(* Logix 5000 AddOnInstructionDefinition export Banner_Q4X_Param_v4; software revision 33.00 *)

TYPE Banner_IOL_Port_v4 :   // UDT that has all of the data items necessary to communicate with a specific Port on a IO-Link Master
STRUCT
   Port_Controlled : INT;   // Each bit represents a port on an IO-Link Master. Set to 1 to tell AOI to control that port.
   Port_Activate : INT;   // Each bit represents a port on an IO-Link Master. When ON that port will process any commands in queue.
   Port_Read : INT;   // Each bit represents a port on an IO-Link Master. Used to determine when device AOI has requested a Read command.
   Port_Write : INT;   // Each bit represents a port on an IO-Link Master. Used to determine when device AOI has requested a Write command.
   Port_RW_Complete : INT;   // Each bit represents a port on an IO-Link Master. Tells device AOI that Read or Write request has been completed.
   Port_Device_Read : INT;
   Data_Transfer : SINT[190];   // Array to transfer data from IO-Master to device AOIs.
END_STRUCT
END_TYPE

TYPE Banner_Q4X_RD_v4 :   // UDT that stores the Write Data for a Q4X.
STRUCT
   Master_Cycle_Time : INT;
   Min_Cycle_Time : INT;
   M_Sequence_Capability : INT;
   IO_Link_Version_ID : INT;
   Process_Data_Input_Length : INT;
   Process_Data_Output_Length : INT;
   Combined_Vendor_ID : DINT;   // IO-Link Vendor ID
   Vendor_ID1 : INT;
   Vendor_ID2 : INT;
   Combined_Device_ID : DINT;   // IO-Link Device ID
   Device_ID1 : INT;
   Device_ID2 : INT;
   Device_ID3 : INT;
   Serial_Number : STRING;
   Teach_State : SINT;   // 0 =IDLE, 1 = SP1 Success, 4 = Wait for Command, 5 = Busy, 7 = Error
   SP1_TP1 : SINT;   // 0 = not taught or unsuccessful, 1 = successfully taught
   SP2_TP2 : SINT;   // 0 = not taught or unsuccessful, 1 = successfully taught
   Measurement_Value : DINT;   // Measurement value in .1 mm. Dual mode the value is in percent match to taught object.
   Excess_Gain_Percent : DINT;   // Excess gain expressed as a percentage of minimum signal strength.
   Stability : INT;   // 0 = No target exists, 1 = Marginal or multiple peaks, 2 = Stable
   Multiple_Peak_State : INT;   // 0 = Multiple peaks not present, 1 = Multiple peaks present
   Laser_Fault_Status : INT;   // 0 = Not present, 1 Laser fault present
   BDC1_Totalizer_Counts : DINT;   // Number of totalizer edges seen on BDC1. Range: 0 to 65535.
   BDC2_Totalizer_Counts : DINT;   // Number of totalizer edges seen on BDC2. Range: 0 to 65535.
   Display_String : STRING;   // String currently being displayed on the LED display of the sensor
END_STRUCT
END_TYPE

TYPE Banner_Q4X_v4 :   // All of the parameters for a Q4X.
STRUCT
   Initial_Global_Read : BOOL;   // Determines if all of the IO-Link data has been read into the PLC yet
   Command : INT;   // Value placed in here will activate a read or write to a specifc IO-Link Index
   Read_Data : Banner_Q4X_RD_v4;   // Read Only Data
   Write_Data : Banner_Q4X_WD_v4;   // Write Data
   Archive : Banner_Q4X_WD_v4;   // Archive of Write Data. Used to determine when data needs to be updated in the IO-Link Master.
   Reset : BOOL;   // Resets AOI. This will force a complete parameter read of the sensor.
END_STRUCT
END_TYPE

TYPE Banner_Q4X_WD_v4 :   // UDT that stores the Write Data for a Q4X.
STRUCT
   System_Command : INT;   // See IODD file for list of commands that can be activated via the System Command interface
   Parameter_Access_Lock : SINT;   // Write access to all parameters is prohibited while value is 1. Only this parameter can be adjusted when value is 1.
   Data_Storage_Lock : SINT;   // Automatic data storage is disabled when this value is equal to 1. Read access is not affected.
   Local_Parameterization_Lock : SINT;   // Parameterization via local control elements on device is disabled.
   Local_User_Interface_Lock : SINT;   // Operation of local user interface is disabled.
   Teach_Channel : INT;   // 0 = Default, 1 = BDC1, 2 = BDC2
   BDC1_Setpoint_SP1 : DINT;   // Switch point value in .1 mm increments. Range: varies depending on sensor.
   BDC1_Setpoint_SP2 : DINT;   // In FGS mode defines second switching point parameter. Range: varies depending on sensor.
   BDC1_Swithpoint_Logic : INT;   // 0 = Light Operate, 1 = Dark Operate
   BDC1_BDC_Mode : INT;   // 1 = 1-Pt BGS, 128 = 2-Pt, 129 = Dynamic, 130 = Window or FGS, 131 = Dual
   BDC1_Hysteresis : DINT;   // Should always be 0
   BDC2_Setpoint_SP1 : DINT;   // Switch point value in .1 mm increments. Range: varies depending on sensor.
   BDC2_Setpoint_SP2 : DINT;   // In FGS mode defines second switching point parameter. Range: varies depending on sensor.
   BDC2_Switchpoint_Logic : INT;   // 0 = Light Operate, 1 = Dark Operate
   BDC2_BDC_Mode : INT;   // 1 = 1-Pt BGS, 128 = 2-Pt, 129 = Dynamic, 130 = Window or FGS, 131 = Dual
   BDC2_Hysteresis : DINT;   // Should always be 0
   Response_Speed : INT;   // 0 = 1.5 ms, 1 = 3 ms, 2 = 10 ms, 3 = 25 ms, 4 = 50 ms
   Gain : INT;   // 0 = High excess gain mode, 1 = Standard excess gain mode
   Secondary_Output_Function : INT;   // 0 = Independent Output, 1 = Complimentary Output, 2 = Remote Teach Input, 3 = Laser Off, 4 = Laser On, 5 = Master, 6 = Slave, 7 = Pulse Frequency Modulation
   Zero_Reference_Location : INT;   // 0 = Near, 1 = Far
   Shift_Zero_Reference_After_Teach : INT;   // 0 = On, 1 = Off
   Display_Read : INT;   // 0 = On, 1 = On Inverted, 2 Off, 3 Off Inverted
   Pushbutton_Lockout : INT;   // 0 = No lockout, 1 = Pushbuttons locked, 2 = Operator Lockout
   IOL_Filter_Time : DINT;   // Time to average IOL process data measurement between updates. Range 0 to 65535 ms.
   BDC1_Delay_Mode : INT;   // 0 = Disabled, 1 = On - Off Delay, 2 = Oneshot, 3 = Totalizer
   BDC1_Delay_Timer1 : DINT;   // Time in 1 ms increments for 1.5 and 3 ms response speeds. Time in 10 ms for all other response speeds. If totalizer is selected value is in counts. Range 0 to 9999 ms.
   BDC1_Delay_Timer2 : DINT;   // Off Delay time in 1 ms increments for 1.5 and 3 ms response speeds. Time in 10 ms for all other response speeds. If totalizer is selected value is in counts. Range 0 to 9999 ms.
   BDC1_Teach_Offset_Mode : INT;   // 0 = Auto, 1 = User Selected
   BDC1_Teach_Offset : DINT;   // Teach Offset Mode must be in in User Selected for this to work. After a FGS or BGS teach the setpoint will be offset by the value stored in the parameter. Range: Values vary by sensor.
   BDC1_FGS_Window_Size : DINT;   // Teach Offset Mode must be in User Selected for this to work. Parameter sets the FGS window size. This value create a window +/- the value. Range: Values vary by sensor.
   BDC1_Auto_Thresholding : INT;   // 0 = On, 1 = Off, 2 = High Speed (Dual Mode Only)
   BDC2_Delay_Mode : INT;   // 0 = Disabled, 1 = On - Off Delay, 2 = Oneshot, 3 = Totalizer
   BDC2_Delay_Timer1 : DINT;   // Time in 1 ms increments for 1.5 and 3 ms response speeds. Time in 10 ms for all other response speeds. If totalizer is selected value is in counts. Range 0 to 9999 ms.
   BDC2_Delay_Timer2 : DINT;   // Off Delay time in 1 ms increments for 1.5 and 3 ms response speeds. Time in 10 ms for all other response speeds. If totalizer is selected value is in counts. Range 0 to 9999 ms.
   BDC2_Teach_Offset_Mode : INT;   // 0 = Auto, 1 = User Selected
   BDC2_Teach_Offset : DINT;   // Teach Offset Mode must be in in User Selected for this to work. After a FGS or BGS teach the setpoint will be offset by the value stored in the parameter. Range: Values vary by sensor.
   BDC2_FGS_Window_Size : DINT;   // Teach Offset Mode must be in User Selected for this to work. Parameter sets the FGS window size. This value create a window +/- the value. Range: Values vary by sensor.
   BDC2_Auto_Thresholding : INT;   // 0 = On, 1 = Off, 2 = High Speed (Dual Mode Only)
   Near_Frequency : DINT;   // Frequency corresponding to a target at the near limit of the sensing range. Range 10 to 45000 Hz.
   Far_Frequency : DINT;   // Frequency corresponding to a target at the far limit of the sensing range. Range 10 to 45000 Hz.
END_STRUCT
END_TYPE

ADD_ON_INSTRUCTION Banner_Q4X_Param_v4   (* revision 4.2, vendor Banner Engineering *)
// AOI to read and write parameter data to an IO-Link Q4X.
// Revision note:
// Fixed an issue with the Device ID parameter.
VAR_IN_OUT
   Q4X : Banner_Q4X_v4; {required}
   Port_Data : Banner_IOL_Port_v4; {required}
END_VAR
VAR_INPUT
   Port : INT; {required}   // Enter the Port number that this AOI is to work with.
END_VAR
VAR
   Local_Control : DINT; {access None}
   Global_Read_Command_Value : INT; {access None}
   Global_Write_Command_Value : INT; {access None}
   Command_Being_Processed : BOOL; {access None}
   Update_Archive : BOOL; {access None}
   Index_Write_Inprocess : INT; {access None}
   Index_Write_Control : INT; {access None}
   Temp_Excess_Gain : DINT[2]; {access None}
   Inprocess_Index : DINT; {access None}
END_VAR

ROUTINE Logic   (* ladder *)
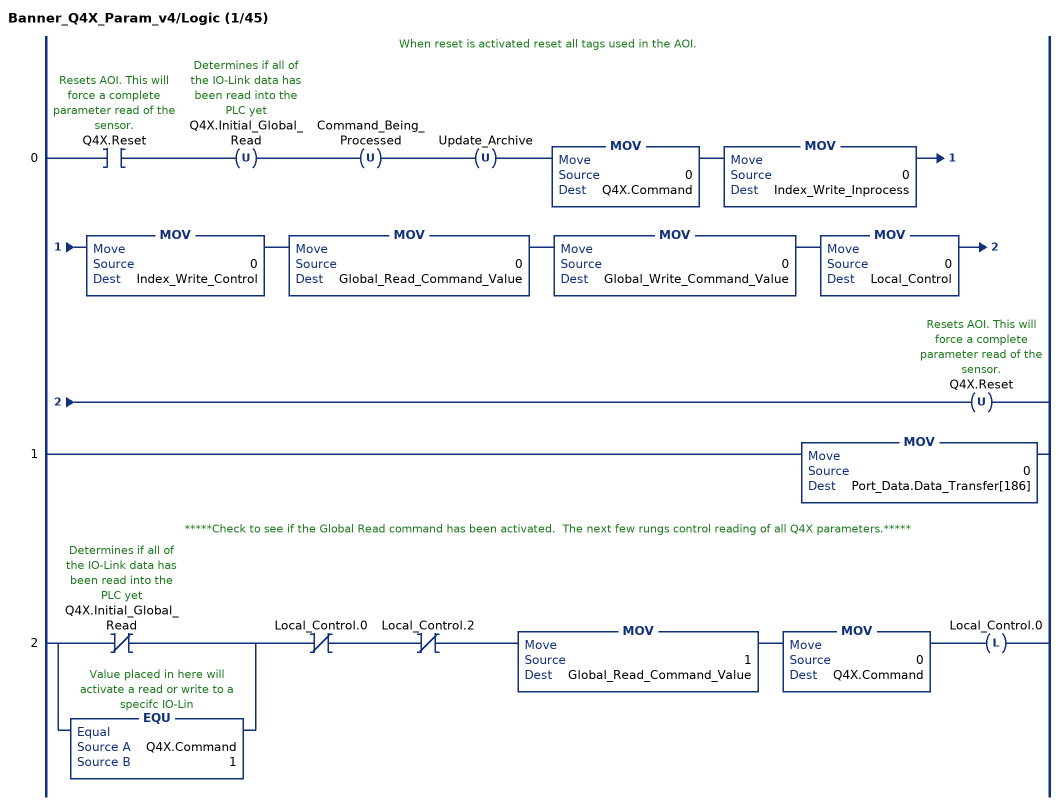
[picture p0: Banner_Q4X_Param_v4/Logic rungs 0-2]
   // When reset is activated reset all tags used in the AOI.
   0: XIC(Q4X.Reset)OTU(Q4X.Initial_Global_Read)OTU(Command_Being_Processed)OTU(Update_Archive)MOV(0,Q4X.Command)MOV(0,Index_Write_Inprocess)MOV(0,Index_Write_Control)MOV(0,Global_Read_Command_Value)MOV(0,Global_Write_Command_Value)MOV(0,Local_Control)OTU(Q4X.Reset);
   1: MOV(0,Port_Data.Data_Transfer[186]);
   // *****Check to see if the Global Read command has been activated.  The next few rungs control reading of all Q4X parameters.*****
   2: [XIO(Q4X.Initial_Global_Read) ,EQU(Q4X.Command,1) ]XIO(Local_Control.0)XIO(Local_Control.2)MOV(1,Global_Read_Command_Value)MOV(0,Q4X.Command)OTL(Local_Control.0);
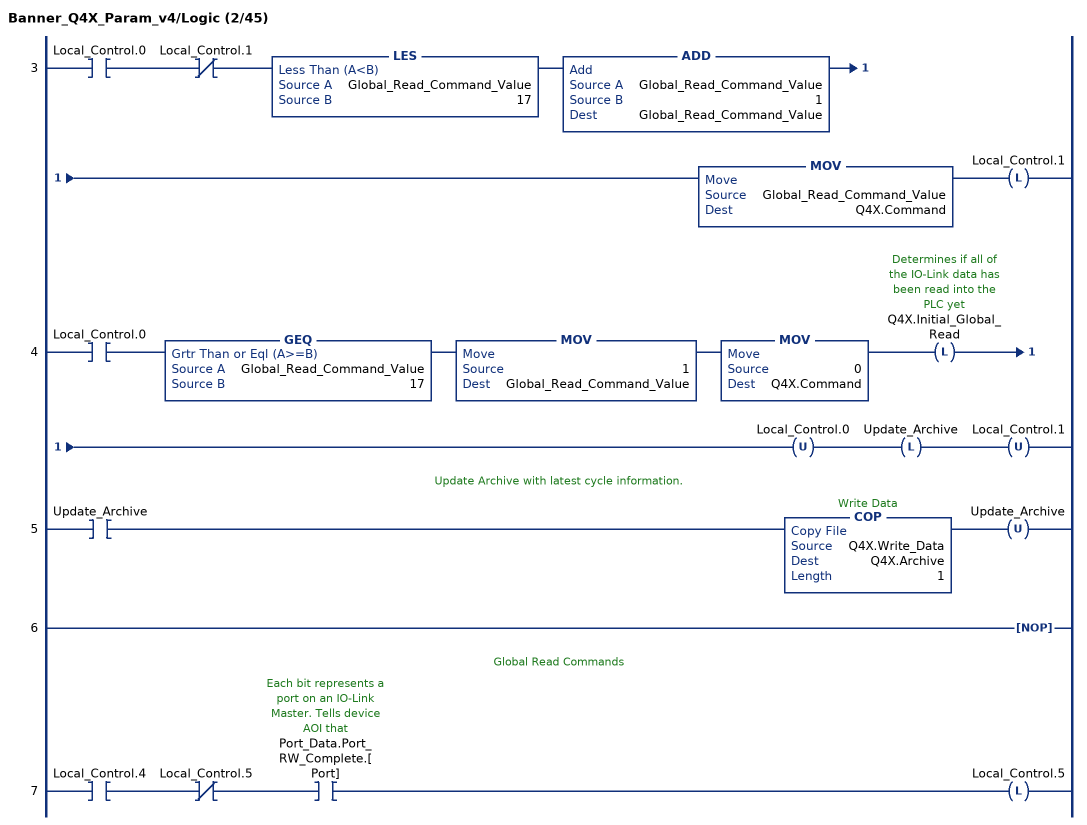
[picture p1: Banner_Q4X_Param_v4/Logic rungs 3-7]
   3: XIC(Local_Control.0)XIO(Local_Control.1)LES(Global_Read_Command_Value,17)ADD(Global_Read_Command_Value,1,Global_Read_Command_Value)MOV(Global_Read_Command_Value,Q4X.Command)OTL(Local_Control.1);
   4: XIC(Local_Control.0)GEQ(Global_Read_Command_Value,17)MOV(1,Global_Read_Command_Value)MOV(0,Q4X.Command)OTL(Q4X.Initial_Global_Read)OTU(Local_Control.0)OTL(Update_Archive)OTU(Local_Control.1);
   // Update Archive with latest cycle information.
   5: XIC(Update_Archive)COP(Q4X.Write_Data,Q4X.Archive,1)OTU(Update_Archive);
   6: NOP();
   // Global Read Commands
   7: XIC(Local_Control.4)XIO(Local_Control.5)XIC(Port_Data.Port_RW_Complete.[Port])OTL(Local_Control.5);
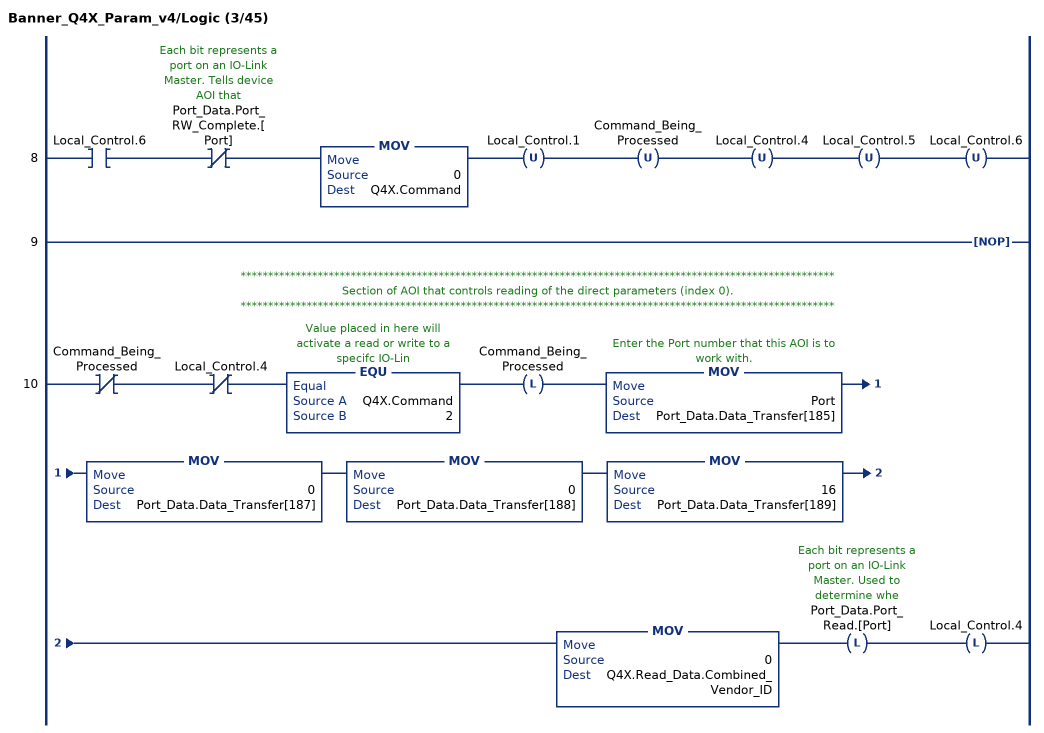
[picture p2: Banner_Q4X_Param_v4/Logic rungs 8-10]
   8: XIC(Local_Control.6)XIO(Port_Data.Port_RW_Complete.[Port])MOV(0,Q4X.Command)OTU(Local_Control.1)OTU(Command_Being_Processed)OTU(Local_Control.4)OTU(Local_Control.5)OTU(Local_Control.6);
   9: NOP();
   // ************************************************************************************************************
   // Section of AOI that controls reading of the direct parameters (index 0).
   // ************************************************************************************************************
   10: XIO(Command_Being_Processed)XIO(Local_Control.4)EQU(Q4X.Command,2)OTL(Command_Being_Processed)MOV(Port,Port_Data.Data_Transfer[185])MOV(0,Port_Data.Data_Transfer[187])MOV(0,Port_Data.Data_Transfer[188])MOV(16,Port_Data.Data_Transfer[189])MOV(0,Q4X.Read_Data.Combined_Vendor_ID)OTL(Port_Data.Port_Read.[Port])OTL(Local_Control.4);
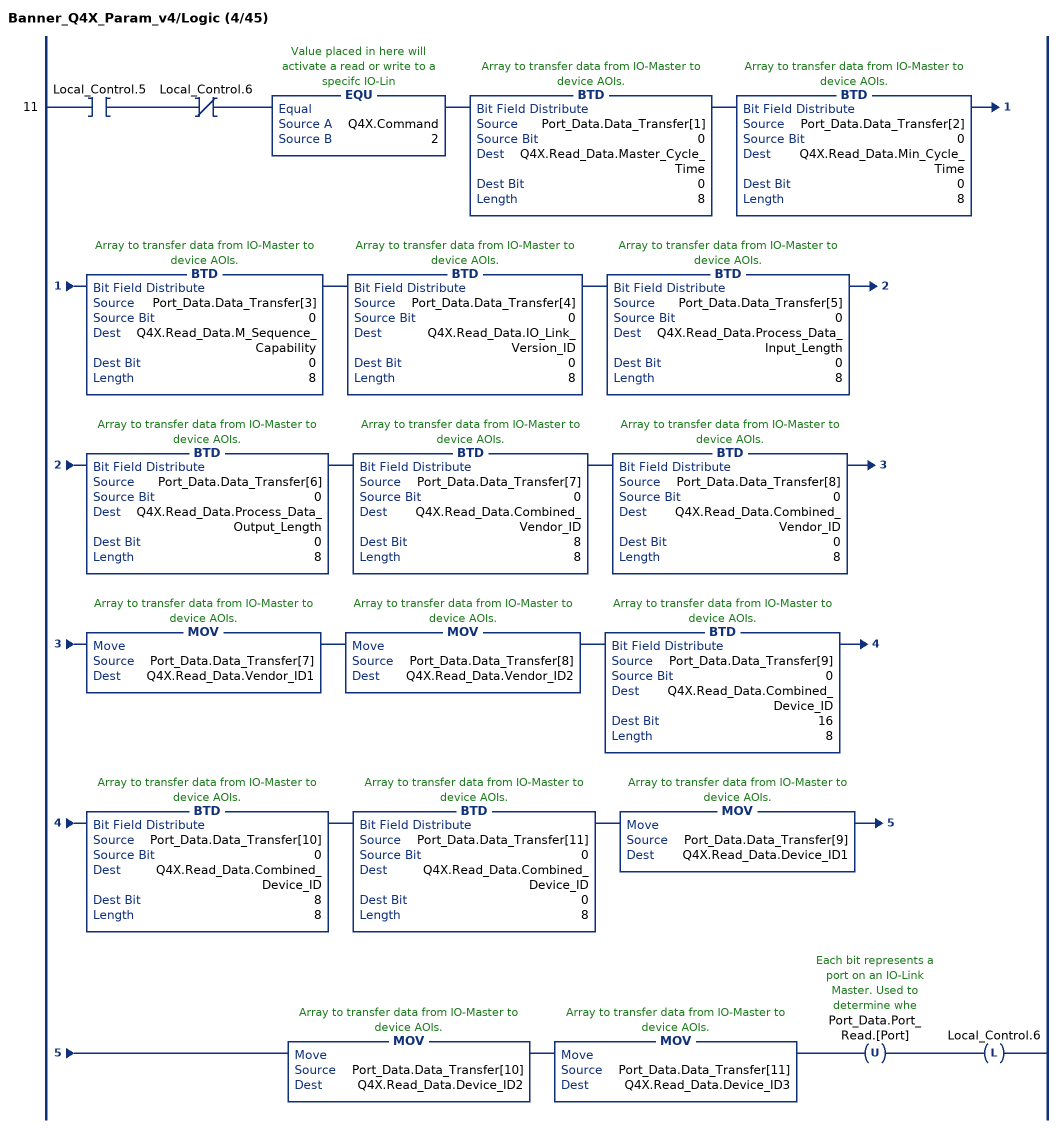
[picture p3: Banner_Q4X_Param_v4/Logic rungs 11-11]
   11: XIC(Local_Control.5)XIO(Local_Control.6)EQU(Q4X.Command,2)BTD(Port_Data.Data_Transfer[1],0,Q4X.Read_Data.Master_Cycle_Time,0,8)BTD(Port_Data.Data_Transfer[2],0,Q4X.Read_Data.Min_Cycle_Time,0,8)BTD(Port_Data.Data_Transfer[3],0,Q4X.Read_Data.M_Sequence_Capability,0,8)BTD(Port_Data.Data_Transfer[4],0,Q4X.Read_Data.IO_Link_Version_ID,0,8)BTD(Port_Data.Data_Transfer[5],0,Q4X.Read_Data.Process_Data_Input_Length,0,8)BTD(Port_Data.Data_Transfer[6],0,Q4X.Read_Data.Process_Data_Output_Length,0,8)BTD(Port_Data.Data_Transfer[7],0,Q4X.Read_Data.Combined_Vendor_ID,8,8)BTD(Port_Data.Data_Transfer[8],0,Q4X.Read_Data.Combined_Vendor_ID,0,8)MOV(Port_Data.Data_Transfer[7],Q4X.Read_Data.Vendor_ID1)MOV(Port_Data.Data_Transfer[8],Q4X.Read_Data.Vendor_ID2)BTD(Port_Data.Data_Transfer[9],0,Q4X.Read_Data.Combined_Device_ID,16,8)BTD(Port_Data.Data_Transfer[10],0,Q4X.Read_Data.Combined_Device_ID,8,8)BTD(Port_Data.Data_Transfer[11],0,Q4X.Read_Data.Combined_Device_ID,0,8)MOV(Port_Data.Data_Transfer[9],Q4X.Read_Data.Device_ID1)MOV(Port_Data.Data_Transfer[10],Q4X.Read_Data.Device_ID2)MOV(Port_Data.Data_Transfer[11],Q4X.Read_Data.Device_ID3)OTU(Port_Data.Port_Read.[Port])OTL(Local_Control.6);
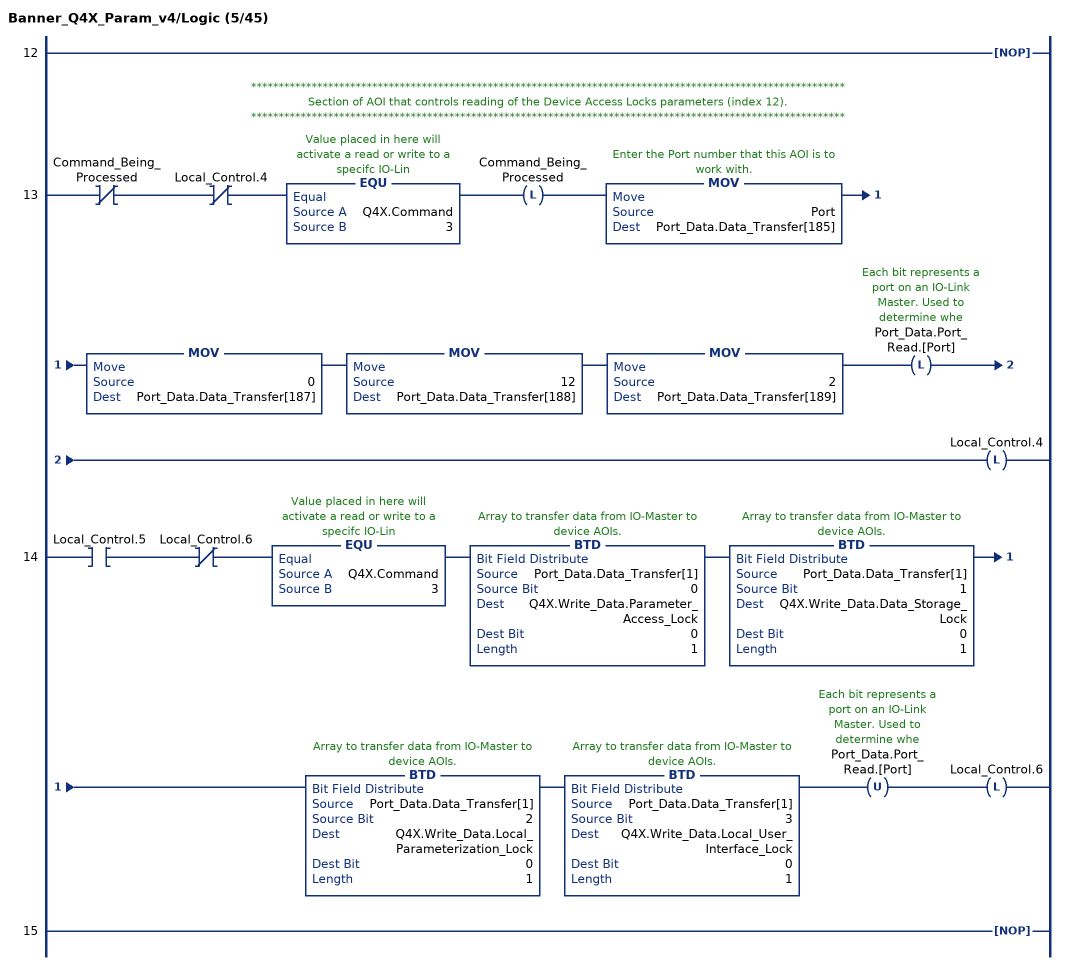
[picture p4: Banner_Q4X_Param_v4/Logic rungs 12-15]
   12: NOP();
   // ************************************************************************************************************
   // Section of AOI that controls reading of the Device Access Locks parameters (index 12).
   // ************************************************************************************************************
   13: XIO(Command_Being_Processed)XIO(Local_Control.4)EQU(Q4X.Command,3)OTL(Command_Being_Processed)MOV(Port,Port_Data.Data_Transfer[185])MOV(0,Port_Data.Data_Transfer[187])MOV(12,Port_Data.Data_Transfer[188])MOV(2,Port_Data.Data_Transfer[189])OTL(Port_Data.Port_Read.[Port])OTL(Local_Control.4);
   14: XIC(Local_Control.5)XIO(Local_Control.6)EQU(Q4X.Command,3)BTD(Port_Data.Data_Transfer[1],0,Q4X.Write_Data.Parameter_Access_Lock,0,1)BTD(Port_Data.Data_Transfer[1],1,Q4X.Write_Data.Data_Storage_Lock,0,1)BTD(Port_Data.Data_Transfer[1],2,Q4X.Write_Data.Local_Parameterization_Lock,0,1)BTD(Port_Data.Data_Transfer[1],3,Q4X.Write_Data.Local_User_Interface_Lock,0,1)OTU(Port_Data.Port_Read.[Port])OTL(Local_Control.6);
   15: NOP();
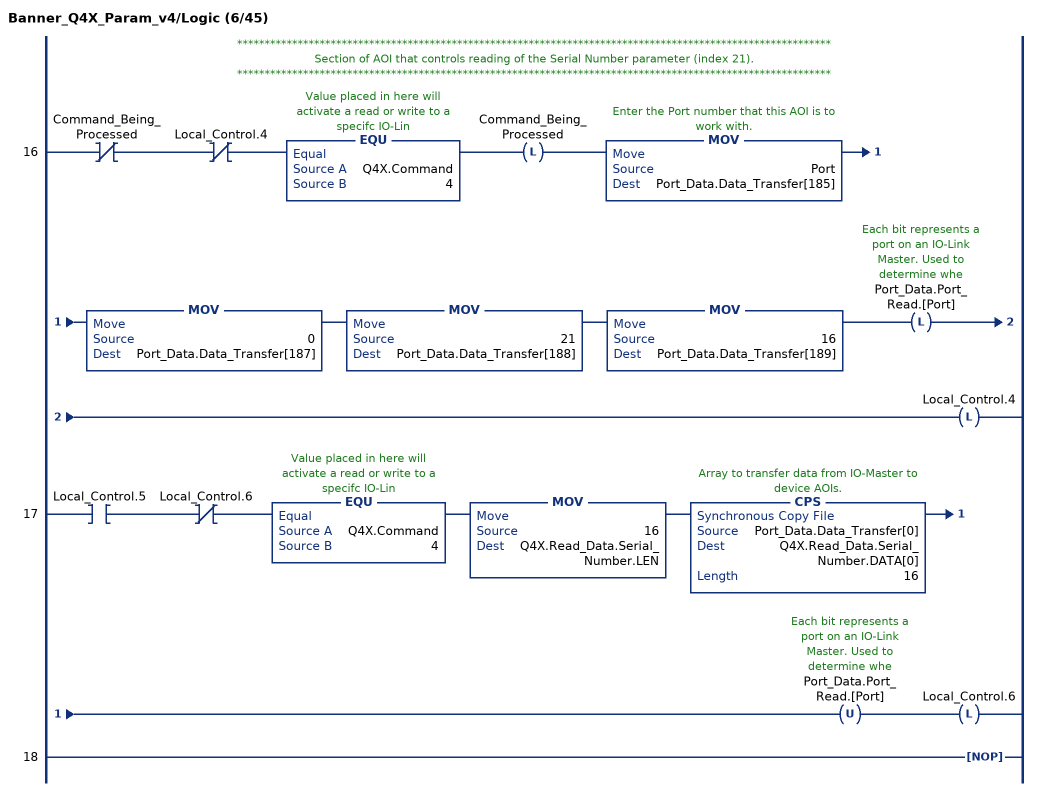
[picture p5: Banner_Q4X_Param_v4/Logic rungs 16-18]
   // ************************************************************************************************************
   // Section of AOI that controls reading of the Serial Number parameter (index 21).
   // ************************************************************************************************************
   16: XIO(Command_Being_Processed)XIO(Local_Control.4)EQU(Q4X.Command,4)OTL(Command_Being_Processed)MOV(Port,Port_Data.Data_Transfer[185])MOV(0,Port_Data.Data_Transfer[187])MOV(21,Port_Data.Data_Transfer[188])MOV(16,Port_Data.Data_Transfer[189])OTL(Port_Data.Port_Read.[Port])OTL(Local_Control.4);
   17: XIC(Local_Control.5)XIO(Local_Control.6)EQU(Q4X.Command,4)MOV(16,Q4X.Read_Data.Serial_Number.LEN)CPS(Port_Data.Data_Transfer[0],Q4X.Read_Data.Serial_Number.DATA[0],16)OTU(Port_Data.Port_Read.[Port])OTL(Local_Control.6);
   18: NOP();
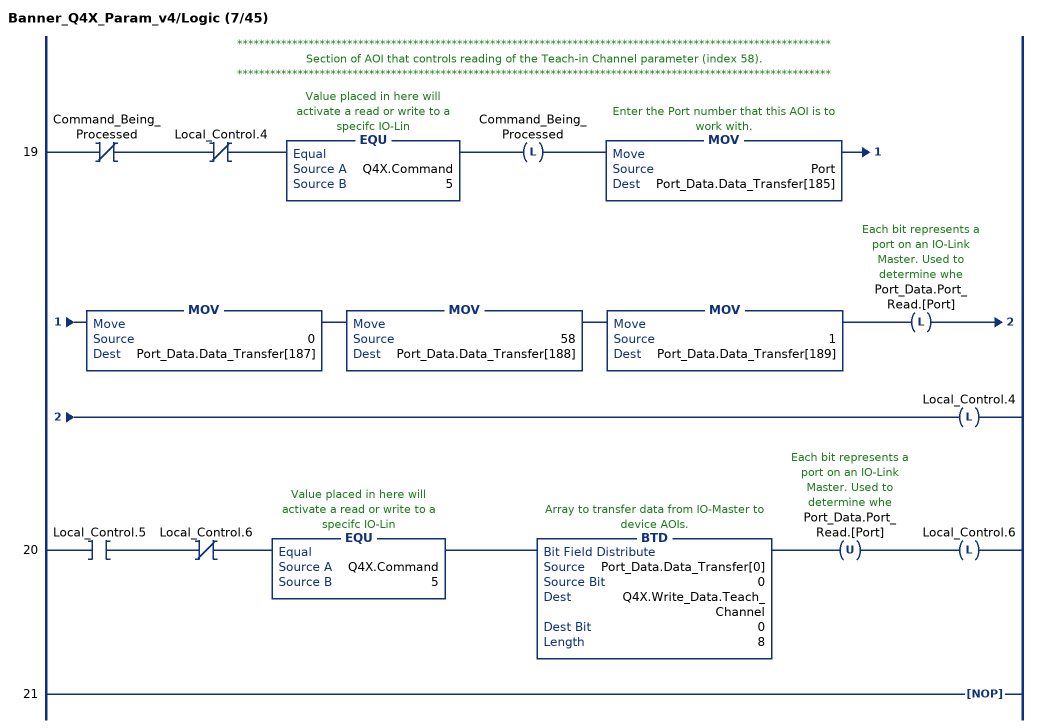
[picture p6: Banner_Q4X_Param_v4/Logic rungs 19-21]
   // ************************************************************************************************************
   // Section of AOI that controls reading of the Teach-in Channel parameter (index 58).
   // ************************************************************************************************************
   19: XIO(Command_Being_Processed)XIO(Local_Control.4)EQU(Q4X.Command,5)OTL(Command_Being_Processed)MOV(Port,Port_Data.Data_Transfer[185])MOV(0,Port_Data.Data_Transfer[187])MOV(58,Port_Data.Data_Transfer[188])MOV(1,Port_Data.Data_Transfer[189])OTL(Port_Data.Port_Read.[Port])OTL(Local_Control.4);
   20: XIC(Local_Control.5)XIO(Local_Control.6)EQU(Q4X.Command,5)BTD(Port_Data.Data_Transfer[0],0,Q4X.Write_Data.Teach_Channel,0,8)OTU(Port_Data.Port_Read.[Port])OTL(Local_Control.6);
   21: NOP();
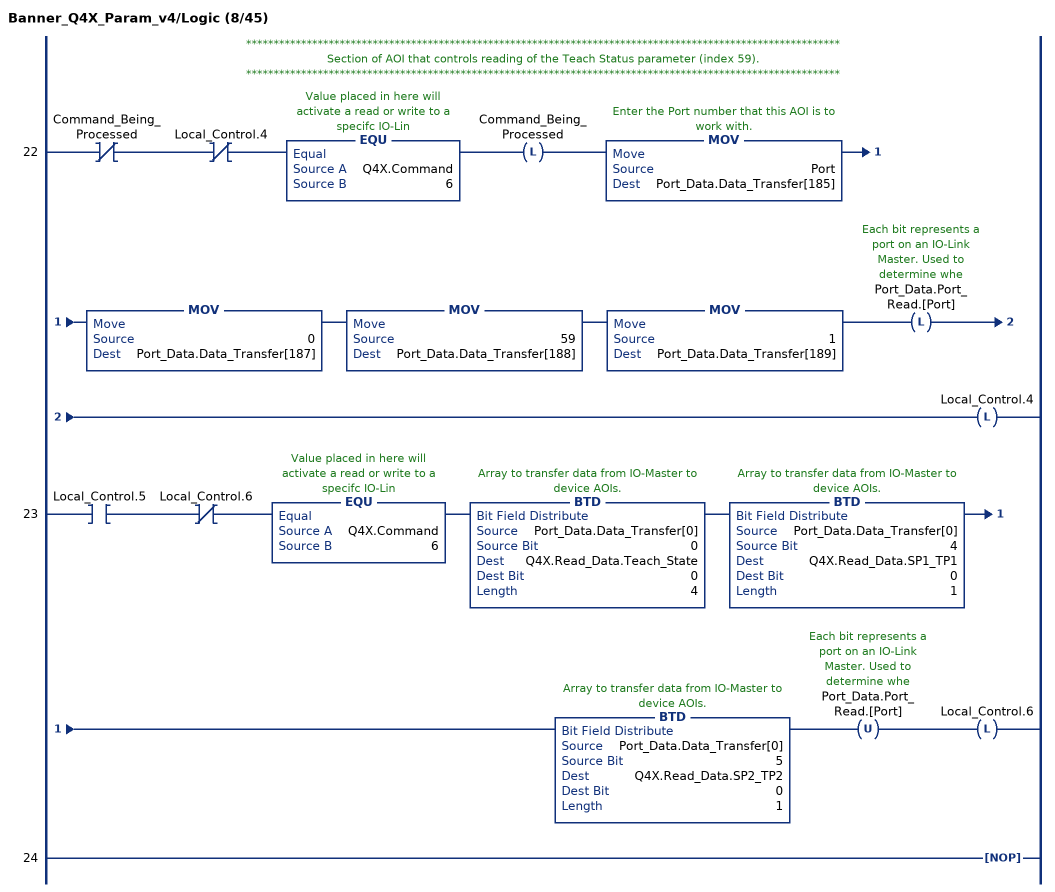
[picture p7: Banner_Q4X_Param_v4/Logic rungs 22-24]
   // ************************************************************************************************************
   // Section of AOI that controls reading of the Teach Status parameter (index 59).
   // ************************************************************************************************************
   22: XIO(Command_Being_Processed)XIO(Local_Control.4)EQU(Q4X.Command,6)OTL(Command_Being_Processed)MOV(Port,Port_Data.Data_Transfer[185])MOV(0,Port_Data.Data_Transfer[187])MOV(59,Port_Data.Data_Transfer[188])MOV(1,Port_Data.Data_Transfer[189])OTL(Port_Data.Port_Read.[Port])OTL(Local_Control.4);
   23: XIC(Local_Control.5)XIO(Local_Control.6)EQU(Q4X.Command,6)BTD(Port_Data.Data_Transfer[0],0,Q4X.Read_Data.Teach_State,0,4)BTD(Port_Data.Data_Transfer[0],4,Q4X.Read_Data.SP1_TP1,0,1)BTD(Port_Data.Data_Transfer[0],5,Q4X.Read_Data.SP2_TP2,0,1)OTU(Port_Data.Port_Read.[Port])OTL(Local_Control.6);
   24: NOP();
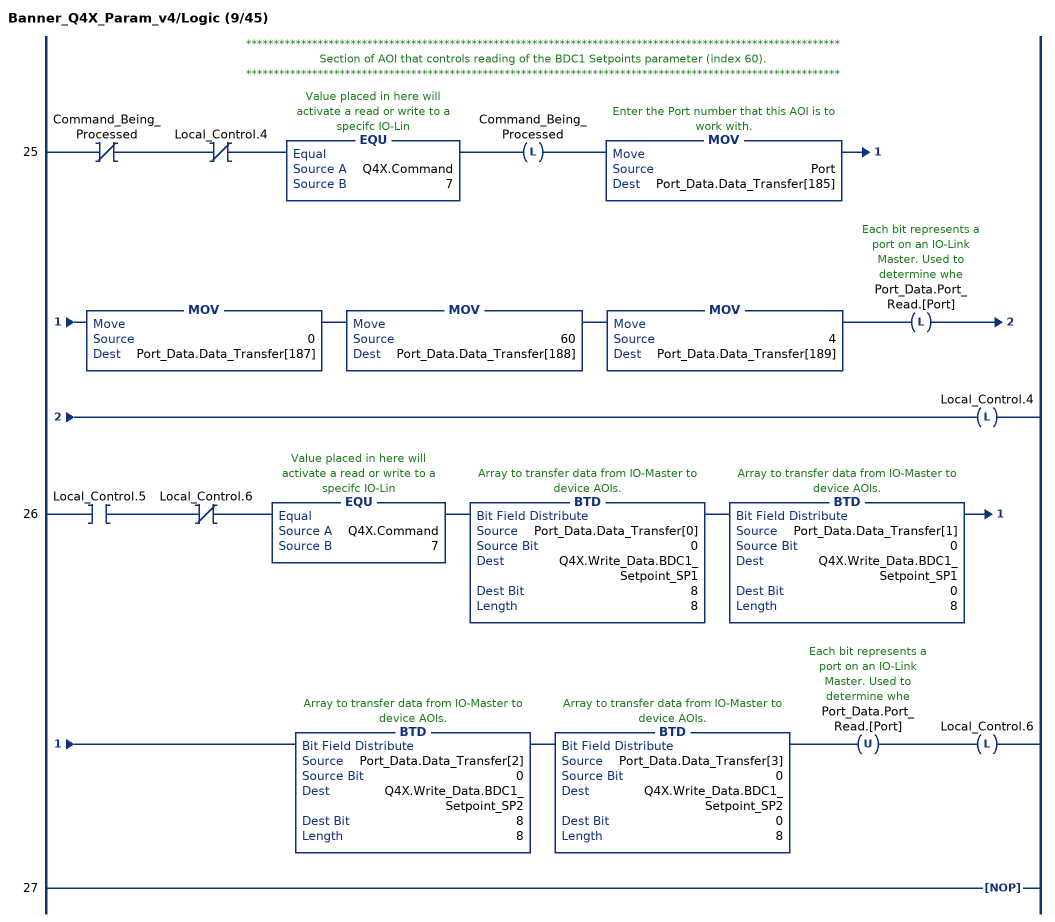
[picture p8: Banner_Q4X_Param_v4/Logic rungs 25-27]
   // ************************************************************************************************************
   // Section of AOI that controls reading of the BDC1 Setpoints parameter (index 60).
   // ************************************************************************************************************
   25: XIO(Command_Being_Processed)XIO(Local_Control.4)EQU(Q4X.Command,7)OTL(Command_Being_Processed)MOV(Port,Port_Data.Data_Transfer[185])MOV(0,Port_Data.Data_Transfer[187])MOV(60,Port_Data.Data_Transfer[188])MOV(4,Port_Data.Data_Transfer[189])OTL(Port_Data.Port_Read.[Port])OTL(Local_Control.4);
   26: XIC(Local_Control.5)XIO(Local_Control.6)EQU(Q4X.Command,7)BTD(Port_Data.Data_Transfer[0],0,Q4X.Write_Data.BDC1_Setpoint_SP1,8,8)BTD(Port_Data.Data_Transfer[1],0,Q4X.Write_Data.BDC1_Setpoint_SP1,0,8)BTD(Port_Data.Data_Transfer[2],0,Q4X.Write_Data.BDC1_Setpoint_SP2,8,8)BTD(Port_Data.Data_Transfer[3],0,Q4X.Write_Data.BDC1_Setpoint_SP2,0,8)OTU(Port_Data.Port_Read.[Port])OTL(Local_Control.6);
   27: NOP();
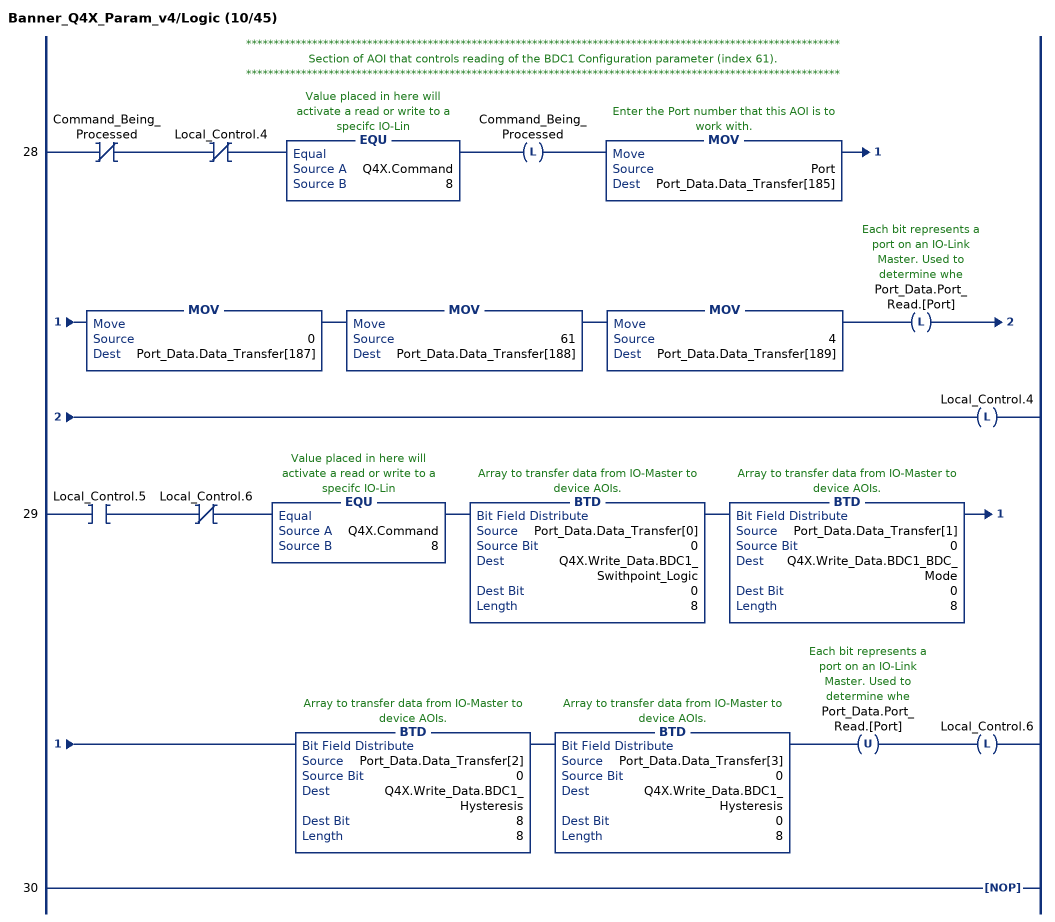
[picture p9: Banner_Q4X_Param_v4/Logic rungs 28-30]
   // ************************************************************************************************************
   // Section of AOI that controls reading of the BDC1 Configuration parameter (index 61).
   // ************************************************************************************************************
   28: XIO(Command_Being_Processed)XIO(Local_Control.4)EQU(Q4X.Command,8)OTL(Command_Being_Processed)MOV(Port,Port_Data.Data_Transfer[185])MOV(0,Port_Data.Data_Transfer[187])MOV(61,Port_Data.Data_Transfer[188])MOV(4,Port_Data.Data_Transfer[189])OTL(Port_Data.Port_Read.[Port])OTL(Local_Control.4);
   29: XIC(Local_Control.5)XIO(Local_Control.6)EQU(Q4X.Command,8)BTD(Port_Data.Data_Transfer[0],0,Q4X.Write_Data.BDC1_Swithpoint_Logic,0,8)BTD(Port_Data.Data_Transfer[1],0,Q4X.Write_Data.BDC1_BDC_Mode,0,8)BTD(Port_Data.Data_Transfer[2],0,Q4X.Write_Data.BDC1_Hysteresis,8,8)BTD(Port_Data.Data_Transfer[3],0,Q4X.Write_Data.BDC1_Hysteresis,0,8)OTU(Port_Data.Port_Read.[Port])OTL(Local_Control.6);
   30: NOP();
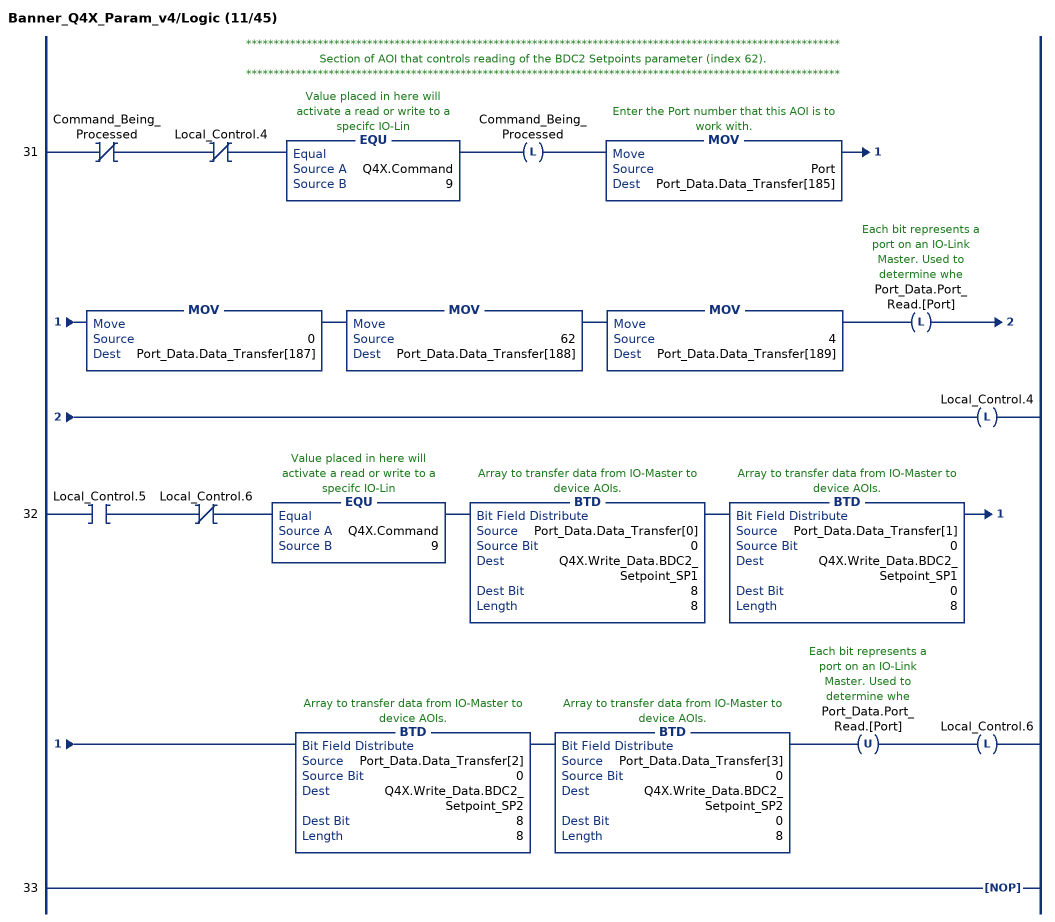
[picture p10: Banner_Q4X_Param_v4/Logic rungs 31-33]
   // ************************************************************************************************************
   // Section of AOI that controls reading of the BDC2 Setpoints parameter (index 62).
   // ************************************************************************************************************
   31: XIO(Command_Being_Processed)XIO(Local_Control.4)EQU(Q4X.Command,9)OTL(Command_Being_Processed)MOV(Port,Port_Data.Data_Transfer[185])MOV(0,Port_Data.Data_Transfer[187])MOV(62,Port_Data.Data_Transfer[188])MOV(4,Port_Data.Data_Transfer[189])OTL(Port_Data.Port_Read.[Port])OTL(Local_Control.4);
   32: XIC(Local_Control.5)XIO(Local_Control.6)EQU(Q4X.Command,9)BTD(Port_Data.Data_Transfer[0],0,Q4X.Write_Data.BDC2_Setpoint_SP1,8,8)BTD(Port_Data.Data_Transfer[1],0,Q4X.Write_Data.BDC2_Setpoint_SP1,0,8)BTD(Port_Data.Data_Transfer[2],0,Q4X.Write_Data.BDC2_Setpoint_SP2,8,8)BTD(Port_Data.Data_Transfer[3],0,Q4X.Write_Data.BDC2_Setpoint_SP2,0,8)OTU(Port_Data.Port_Read.[Port])OTL(Local_Control.6);
   33: NOP();
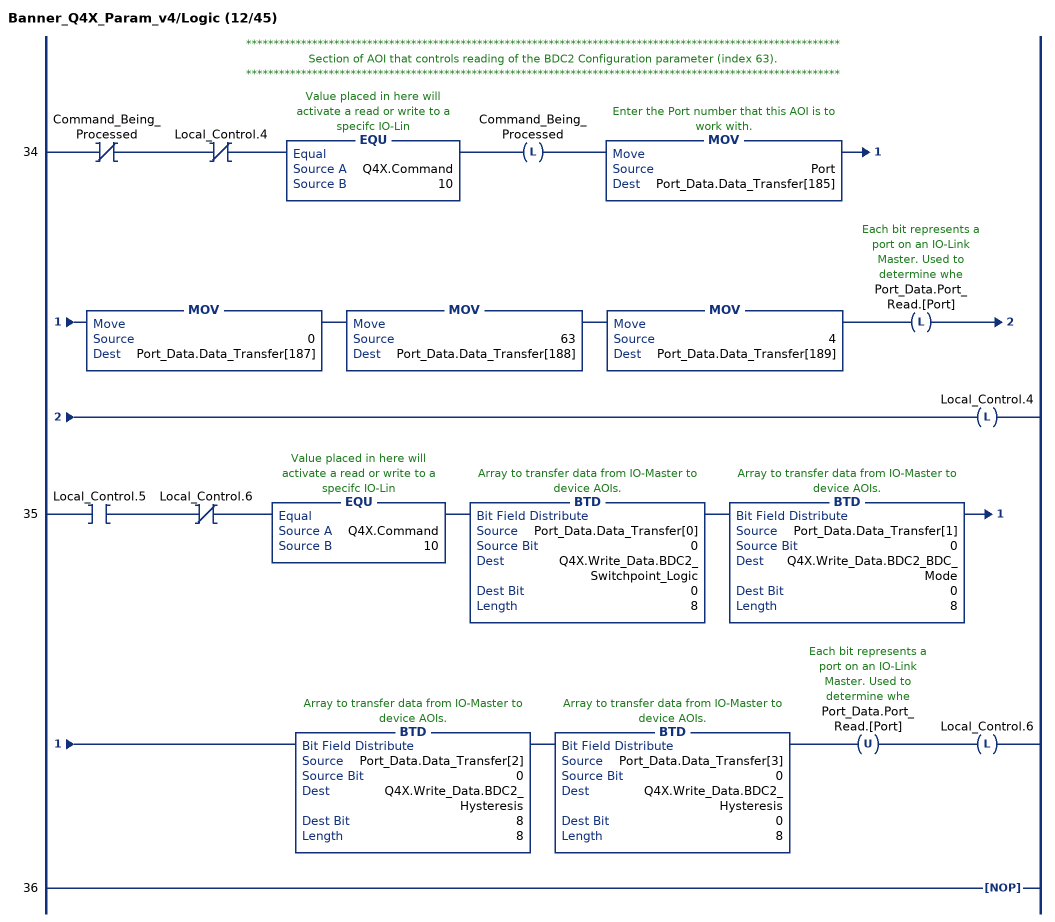
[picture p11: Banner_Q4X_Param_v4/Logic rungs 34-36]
   // ************************************************************************************************************
   // Section of AOI that controls reading of the BDC2 Configuration parameter (index 63).
   // ************************************************************************************************************
   34: XIO(Command_Being_Processed)XIO(Local_Control.4)EQU(Q4X.Command,10)OTL(Command_Being_Processed)MOV(Port,Port_Data.Data_Transfer[185])MOV(0,Port_Data.Data_Transfer[187])MOV(63,Port_Data.Data_Transfer[188])MOV(4,Port_Data.Data_Transfer[189])OTL(Port_Data.Port_Read.[Port])OTL(Local_Control.4);
   35: XIC(Local_Control.5)XIO(Local_Control.6)EQU(Q4X.Command,10)BTD(Port_Data.Data_Transfer[0],0,Q4X.Write_Data.BDC2_Switchpoint_Logic,0,8)BTD(Port_Data.Data_Transfer[1],0,Q4X.Write_Data.BDC2_BDC_Mode,0,8)BTD(Port_Data.Data_Transfer[2],0,Q4X.Write_Data.BDC2_Hysteresis,8,8)BTD(Port_Data.Data_Transfer[3],0,Q4X.Write_Data.BDC2_Hysteresis,0,8)OTU(Port_Data.Port_Read.[Port])OTL(Local_Control.6);
   36: NOP();
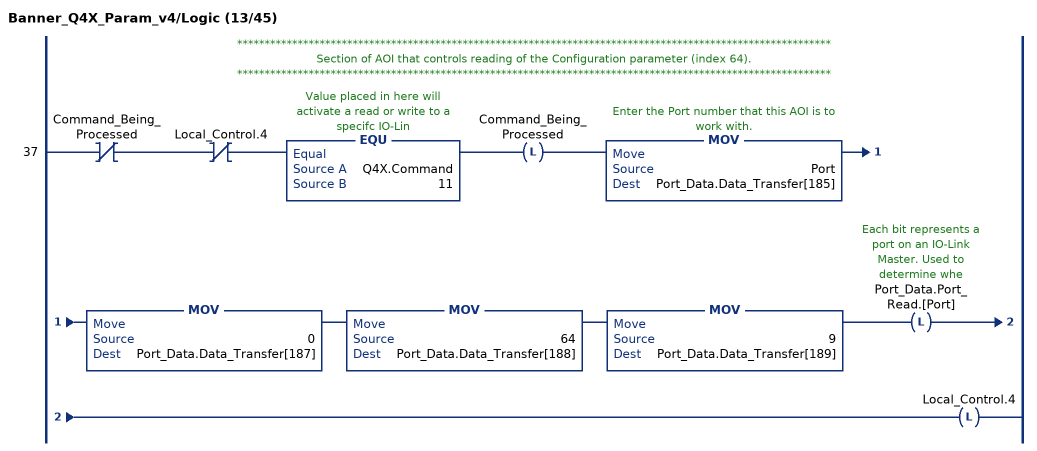
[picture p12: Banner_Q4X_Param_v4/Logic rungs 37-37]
   // ************************************************************************************************************
   // Section of AOI that controls reading of the Configuration parameter (index 64).
   // ************************************************************************************************************
   37: XIO(Command_Being_Processed)XIO(Local_Control.4)EQU(Q4X.Command,11)OTL(Command_Being_Processed)MOV(Port,Port_Data.Data_Transfer[185])MOV(0,Port_Data.Data_Transfer[187])MOV(64,Port_Data.Data_Transfer[188])MOV(9,Port_Data.Data_Transfer[189])OTL(Port_Data.Port_Read.[Port])OTL(Local_Control.4);
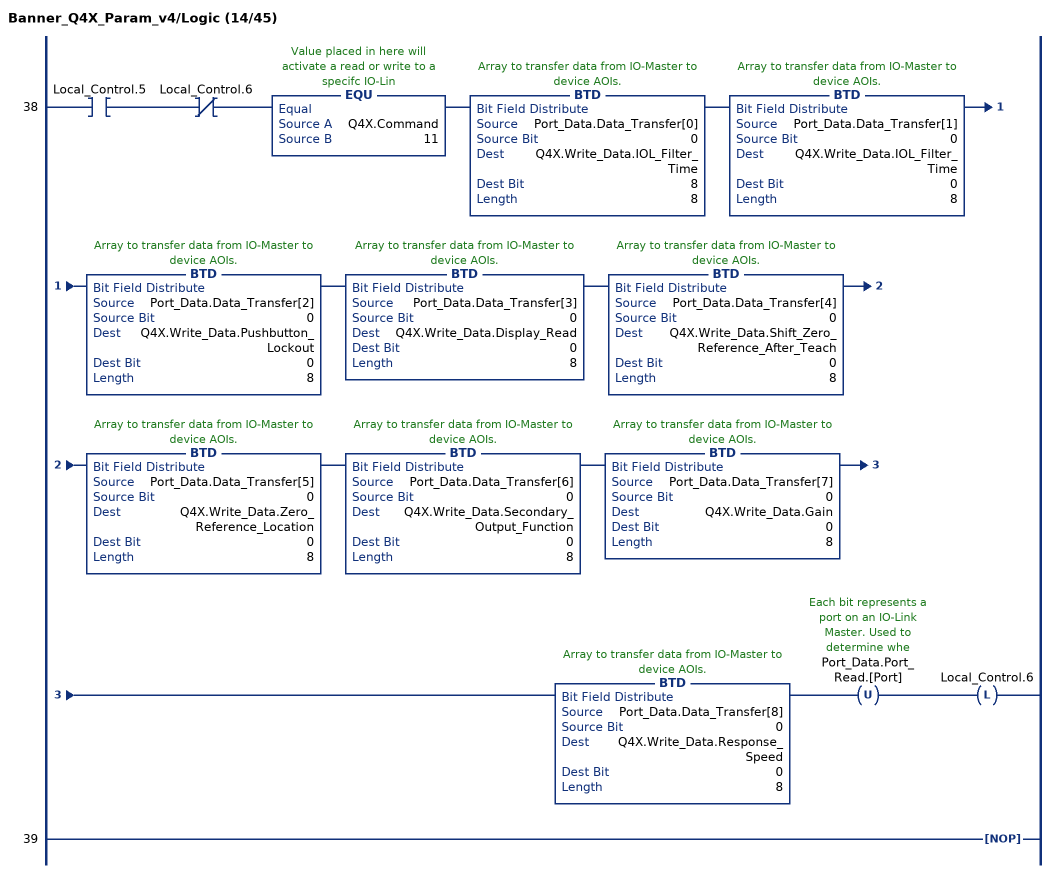
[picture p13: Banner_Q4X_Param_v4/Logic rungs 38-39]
   38: XIC(Local_Control.5)XIO(Local_Control.6)EQU(Q4X.Command,11)BTD(Port_Data.Data_Transfer[0],0,Q4X.Write_Data.IOL_Filter_Time,8,8)BTD(Port_Data.Data_Transfer[1],0,Q4X.Write_Data.IOL_Filter_Time,0,8)BTD(Port_Data.Data_Transfer[2],0,Q4X.Write_Data.Pushbutton_Lockout,0,8)BTD(Port_Data.Data_Transfer[3],0,Q4X.Write_Data.Display_Read,0,8)BTD(Port_Data.Data_Transfer[4],0,Q4X.Write_Data.Shift_Zero_Reference_After_Teach,0,8)BTD(Port_Data.Data_Transfer[5],0,Q4X.Write_Data.Zero_Reference_Location,0,8)BTD(Port_Data.Data_Transfer[6],0,Q4X.Write_Data.Secondary_Output_Function,0,8)BTD(Port_Data.Data_Transfer[7],0,Q4X.Write_Data.Gain,0,8)BTD(Port_Data.Data_Transfer[8],0,Q4X.Write_Data.Response_Speed,0,8)OTU(Port_Data.Port_Read.[Port])OTL(Local_Control.6);
   39: NOP();
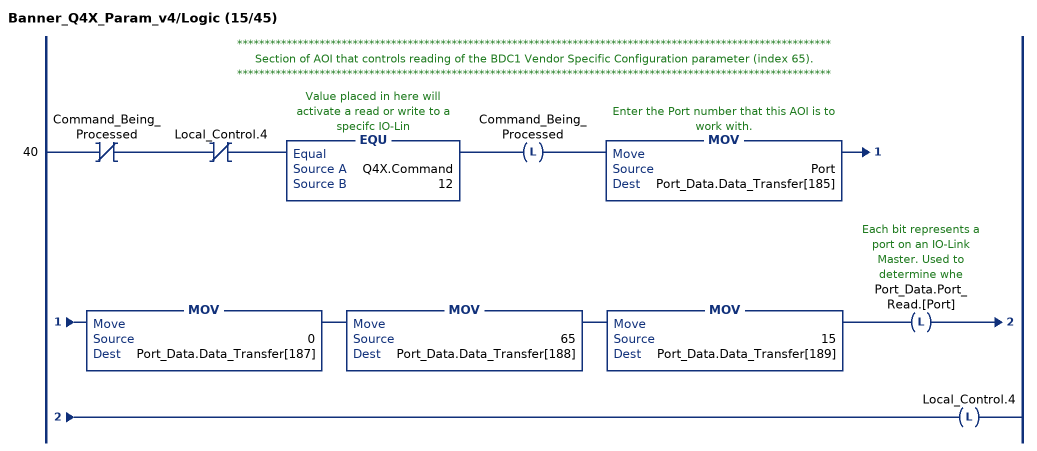
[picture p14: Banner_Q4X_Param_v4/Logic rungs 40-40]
   // ************************************************************************************************************
   // Section of AOI that controls reading of the BDC1 Vendor Specific Configuration parameter (index 65).
   // ************************************************************************************************************
   40: XIO(Command_Being_Processed)XIO(Local_Control.4)EQU(Q4X.Command,12)OTL(Command_Being_Processed)MOV(Port,Port_Data.Data_Transfer[185])MOV(0,Port_Data.Data_Transfer[187])MOV(65,Port_Data.Data_Transfer[188])MOV(15,Port_Data.Data_Transfer[189])OTL(Port_Data.Port_Read.[Port])OTL(Local_Control.4);
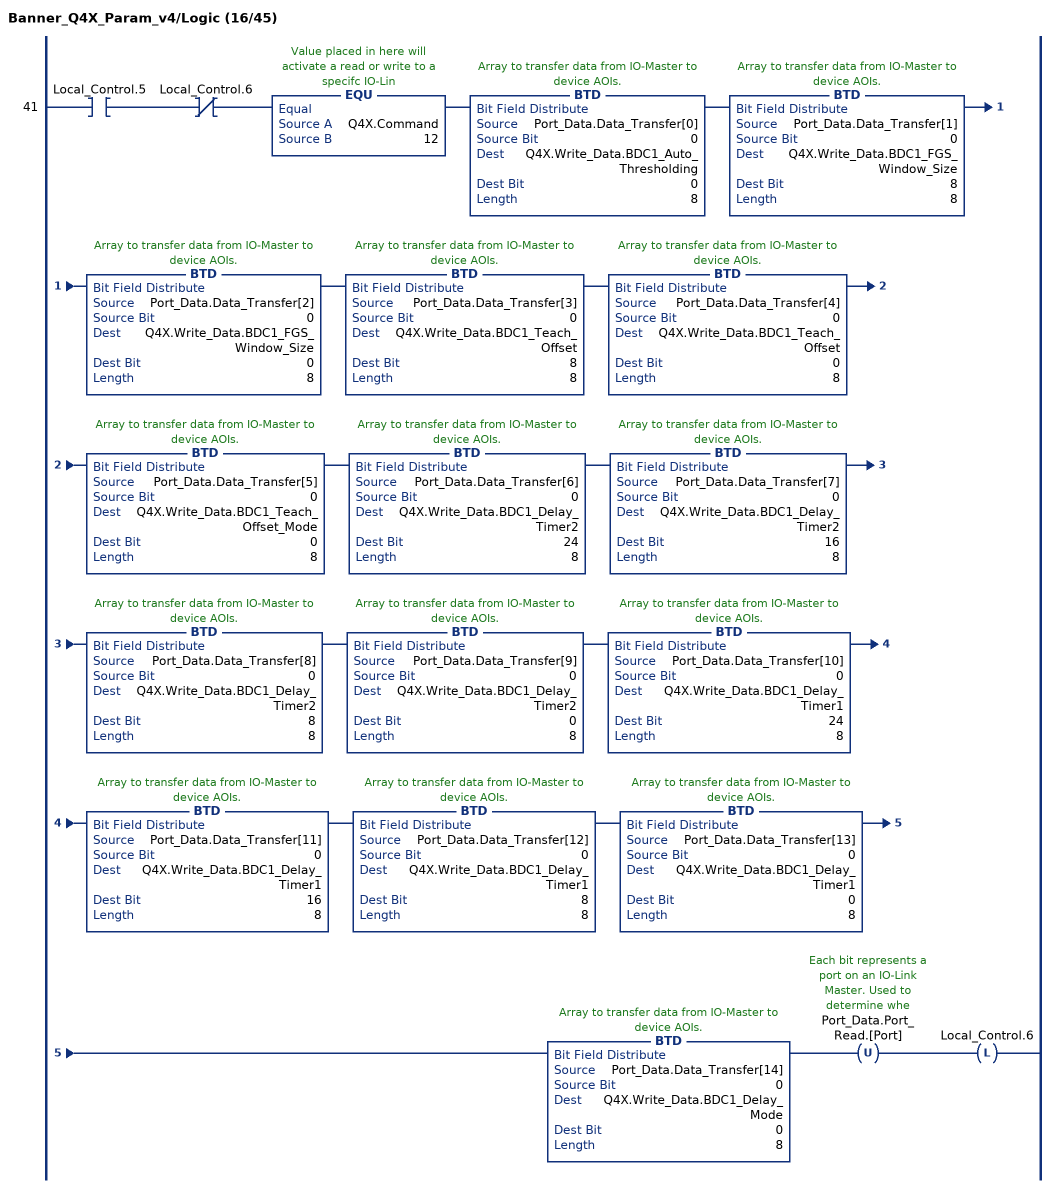
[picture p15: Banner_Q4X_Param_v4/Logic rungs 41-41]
   41: XIC(Local_Control.5)XIO(Local_Control.6)EQU(Q4X.Command,12)BTD(Port_Data.Data_Transfer[0],0,Q4X.Write_Data.BDC1_Auto_Thresholding,0,8)BTD(Port_Data.Data_Transfer[1],0,Q4X.Write_Data.BDC1_FGS_Window_Size,8,8)BTD(Port_Data.Data_Transfer[2],0,Q4X.Write_Data.BDC1_FGS_Window_Size,0,8)BTD(Port_Data.Data_Transfer[3],0,Q4X.Write_Data.BDC1_Teach_Offset,8,8)BTD(Port_Data.Data_Transfer[4],0,Q4X.Write_Data.BDC1_Teach_Offset,0,8)BTD(Port_Data.Data_Transfer[5],0,Q4X.Write_Data.BDC1_Teach_Offset_Mode,0,8)BTD(Port_Data.Data_Transfer[6],0,Q4X.Write_Data.BDC1_Delay_Timer2,24,8)BTD(Port_Data.Data_Transfer[7],0,Q4X.Write_Data.BDC1_Delay_Timer2,16,8)BTD(Port_Data.Data_Transfer[8],0,Q4X.Write_Data.BDC1_Delay_Timer2,8,8)BTD(Port_Data.Data_Transfer[9],0,Q4X.Write_Data.BDC1_Delay_Timer2,0,8)BTD(Port_Data.Data_Transfer[10],0,Q4X.Write_Data.BDC1_Delay_Timer1,24,8)BTD(Port_Data.Data_Transfer[11],0,Q4X.Write_Data.BDC1_Delay_Timer1,16,8)BTD(Port_Data.Data_Transfer[12],0,Q4X.Write_Data.BDC1_Delay_Timer1,8,8)BTD(Port_Data.Data_Transfer[13],0,Q4X.Write_Data.BDC1_Delay_Timer1,0,8)BTD(Port_Data.Data_Transfer[14],0,Q4X.Write_Data.BDC1_Delay_Mode,0,8)OTU(Port_Data.Port_Read.[Port])OTL(Local_Control.6);
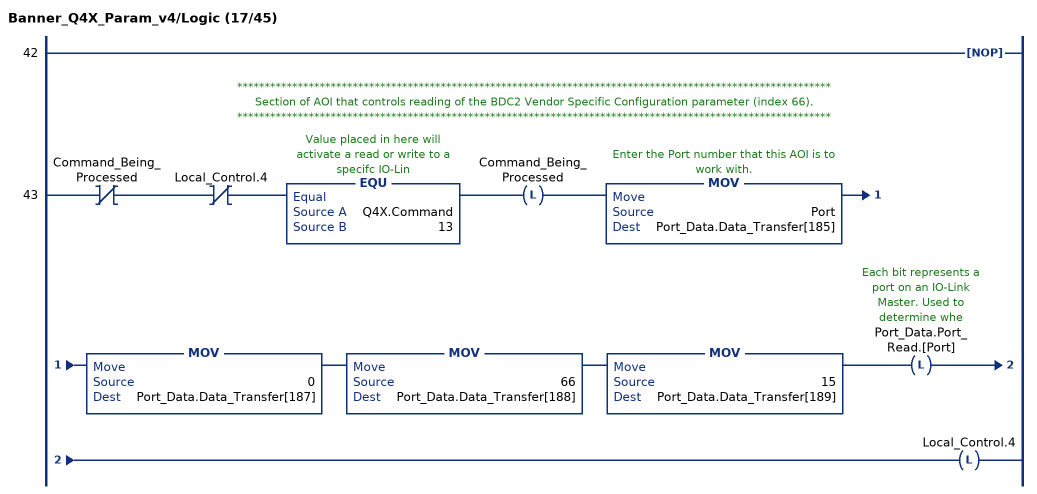
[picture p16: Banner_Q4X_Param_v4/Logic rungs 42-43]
   42: NOP();
   // ************************************************************************************************************
   // Section of AOI that controls reading of the BDC2 Vendor Specific Configuration parameter (index 66).
   // ************************************************************************************************************
   43: XIO(Command_Being_Processed)XIO(Local_Control.4)EQU(Q4X.Command,13)OTL(Command_Being_Processed)MOV(Port,Port_Data.Data_Transfer[185])MOV(0,Port_Data.Data_Transfer[187])MOV(66,Port_Data.Data_Transfer[188])MOV(15,Port_Data.Data_Transfer[189])OTL(Port_Data.Port_Read.[Port])OTL(Local_Control.4);
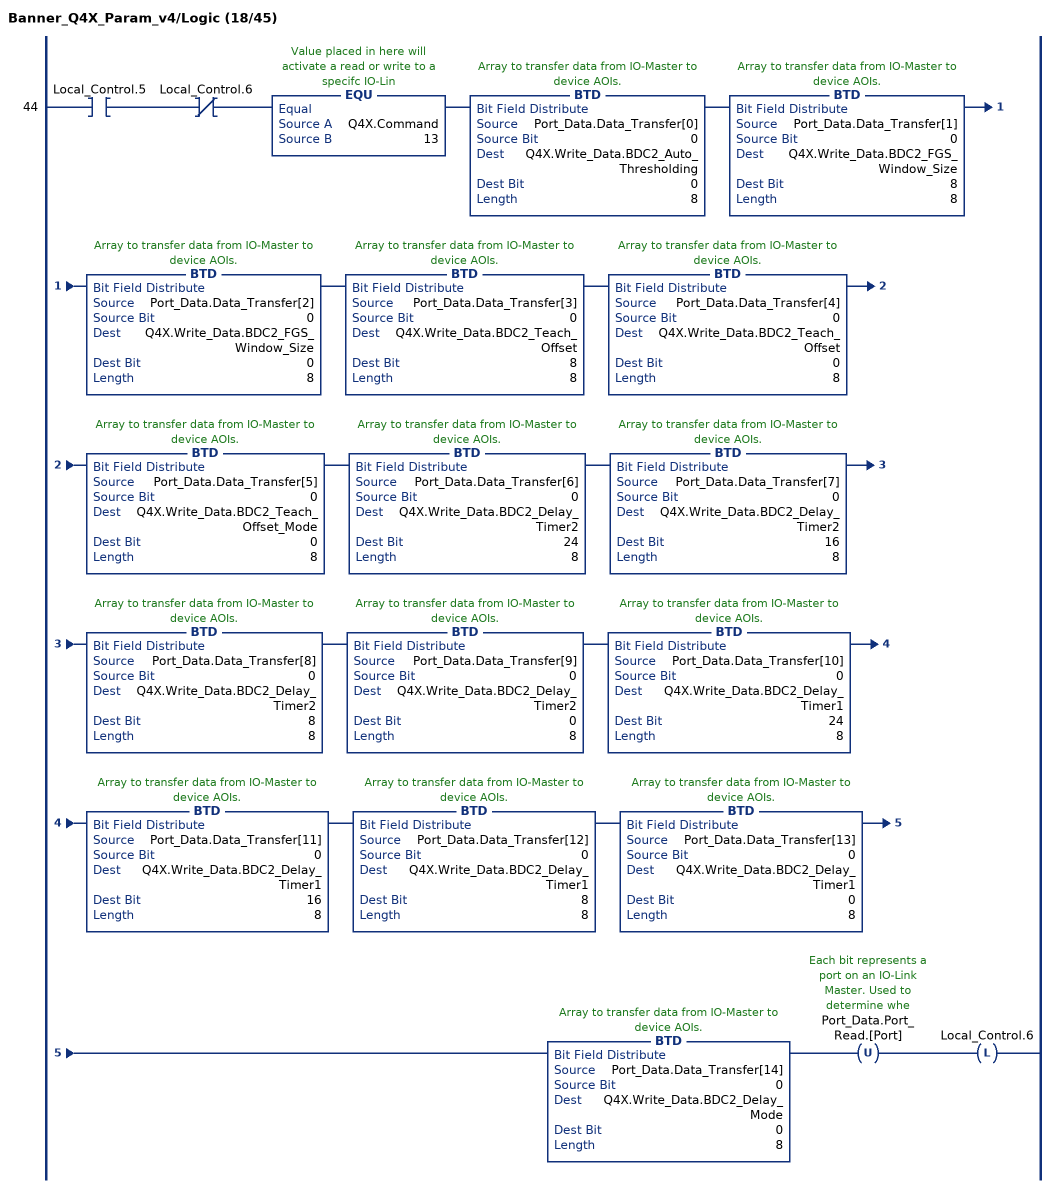
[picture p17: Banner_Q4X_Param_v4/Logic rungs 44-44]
   44: XIC(Local_Control.5)XIO(Local_Control.6)EQU(Q4X.Command,13)BTD(Port_Data.Data_Transfer[0],0,Q4X.Write_Data.BDC2_Auto_Thresholding,0,8)BTD(Port_Data.Data_Transfer[1],0,Q4X.Write_Data.BDC2_FGS_Window_Size,8,8)BTD(Port_Data.Data_Transfer[2],0,Q4X.Write_Data.BDC2_FGS_Window_Size,0,8)BTD(Port_Data.Data_Transfer[3],0,Q4X.Write_Data.BDC2_Teach_Offset,8,8)BTD(Port_Data.Data_Transfer[4],0,Q4X.Write_Data.BDC2_Teach_Offset,0,8)BTD(Port_Data.Data_Transfer[5],0,Q4X.Write_Data.BDC2_Teach_Offset_Mode,0,8)BTD(Port_Data.Data_Transfer[6],0,Q4X.Write_Data.BDC2_Delay_Timer2,24,8)BTD(Port_Data.Data_Transfer[7],0,Q4X.Write_Data.BDC2_Delay_Timer2,16,8)BTD(Port_Data.Data_Transfer[8],0,Q4X.Write_Data.BDC2_Delay_Timer2,8,8)BTD(Port_Data.Data_Transfer[9],0,Q4X.Write_Data.BDC2_Delay_Timer2,0,8)BTD(Port_Data.Data_Transfer[10],0,Q4X.Write_Data.BDC2_Delay_Timer1,24,8)BTD(Port_Data.Data_Transfer[11],0,Q4X.Write_Data.BDC2_Delay_Timer1,16,8)BTD(Port_Data.Data_Transfer[12],0,Q4X.Write_Data.BDC2_Delay_Timer1,8,8)BTD(Port_Data.Data_Transfer[13],0,Q4X.Write_Data.BDC2_Delay_Timer1,0,8)BTD(Port_Data.Data_Transfer[14],0,Q4X.Write_Data.BDC2_Delay_Mode,0,8)OTU(Port_Data.Port_Read.[Port])OTL(Local_Control.6);
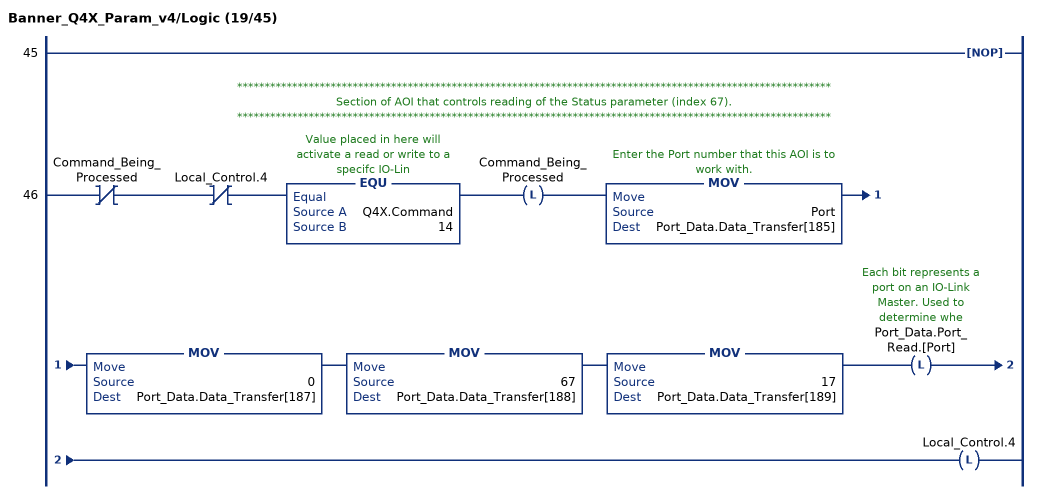
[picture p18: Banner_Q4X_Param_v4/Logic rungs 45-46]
   45: NOP();
   // ************************************************************************************************************
   // Section of AOI that controls reading of the Status parameter (index 67).
   // ************************************************************************************************************
   46: XIO(Command_Being_Processed)XIO(Local_Control.4)EQU(Q4X.Command,14)OTL(Command_Being_Processed)MOV(Port,Port_Data.Data_Transfer[185])MOV(0,Port_Data.Data_Transfer[187])MOV(67,Port_Data.Data_Transfer[188])MOV(17,Port_Data.Data_Transfer[189])OTL(Port_Data.Port_Read.[Port])OTL(Local_Control.4);
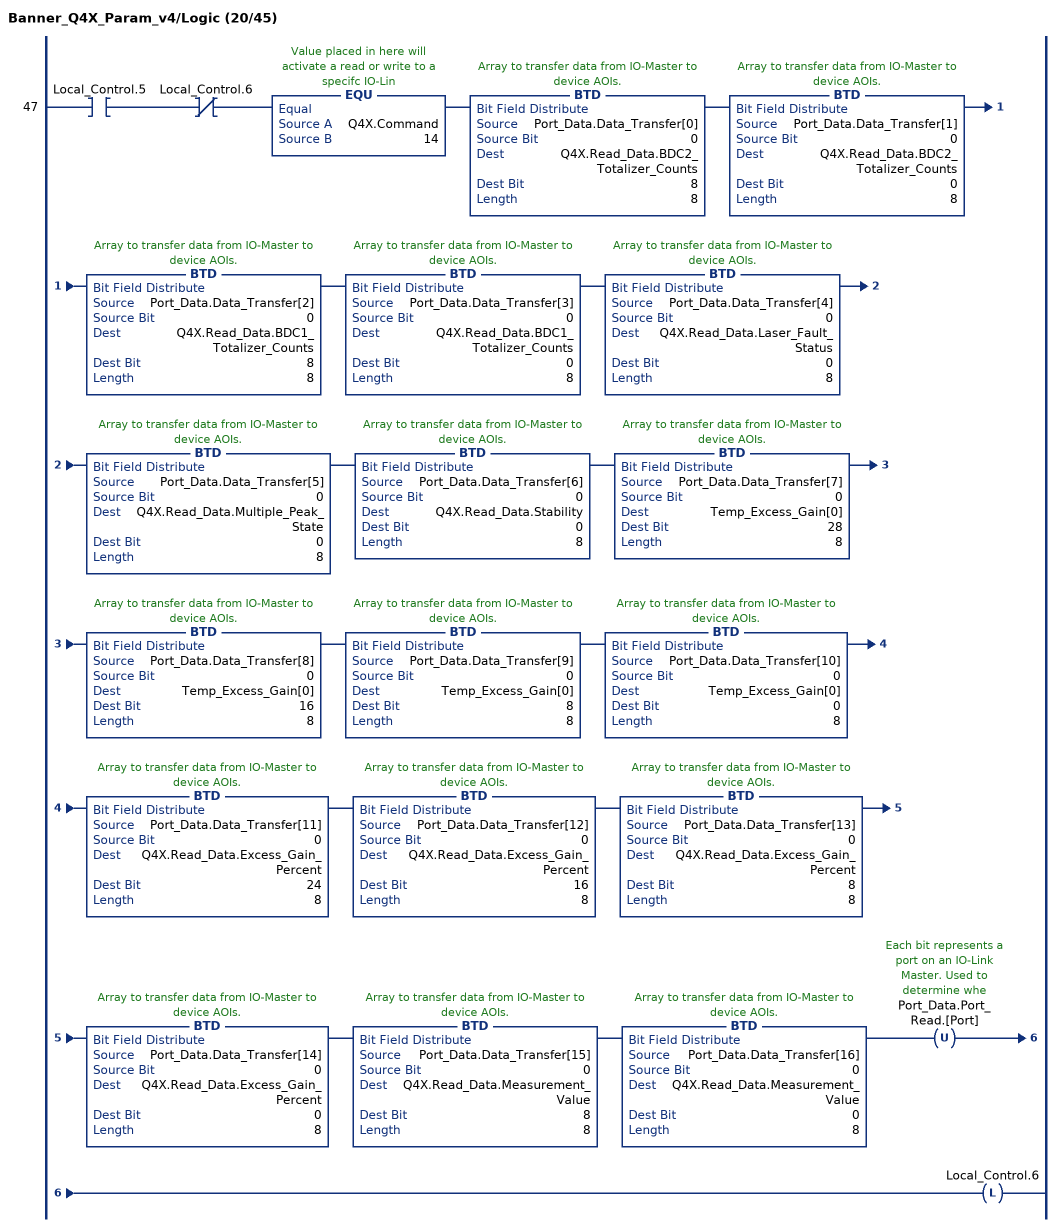
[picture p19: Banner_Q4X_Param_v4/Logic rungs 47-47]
   47: XIC(Local_Control.5)XIO(Local_Control.6)EQU(Q4X.Command,14)BTD(Port_Data.Data_Transfer[0],0,Q4X.Read_Data.BDC2_Totalizer_Counts,8,8)BTD(Port_Data.Data_Transfer[1],0,Q4X.Read_Data.BDC2_Totalizer_Counts,0,8)BTD(Port_Data.Data_Transfer[2],0,Q4X.Read_Data.BDC1_Totalizer_Counts,8,8)BTD(Port_Data.Data_Transfer[3],0,Q4X.Read_Data.BDC1_Totalizer_Counts,0,8)BTD(Port_Data.Data_Transfer[4],0,Q4X.Read_Data.Laser_Fault_Status,0,8)BTD(Port_Data.Data_Transfer[5],0,Q4X.Read_Data.Multiple_Peak_State,0,8)BTD(Port_Data.Data_Transfer[6],0,Q4X.Read_Data.Stability,0,8)BTD(Port_Data.Data_Transfer[7],0,Temp_Excess_Gain[0],28,8)BTD(Port_Data.Data_Transfer[8],0,Temp_Excess_Gain[0],16,8)BTD(Port_Data.Data_Transfer[9],0,Temp_Excess_Gain[0],8,8)BTD(Port_Data.Data_Transfer[10],0,Temp_Excess_Gain[0],0,8)BTD(Port_Data.Data_Transfer[11],0,Q4X.Read_Data.Excess_Gain_Percent,24,8)BTD(Port_Data.Data_Transfer[12],0,Q4X.Read_Data.Excess_Gain_Percent,16,8)BTD(Port_Data.Data_Transfer[13],0,Q4X.Read_Data.Excess_Gain_Percent,8,8)BTD(Port_Data.Data_Transfer[14],0,Q4X.Read_Data.Excess_Gain_Percent,0,8)BTD(Port_Data.Data_Transfer[15],0,Q4X.Read_Data.Measurement_Value,8,8)BTD(Port_Data.Data_Transfer[16],0,Q4X.Read_Data.Measurement_Value,0,8)OTU(Port_Data.Port_Read.[Port])OTL(Local_Control.6);
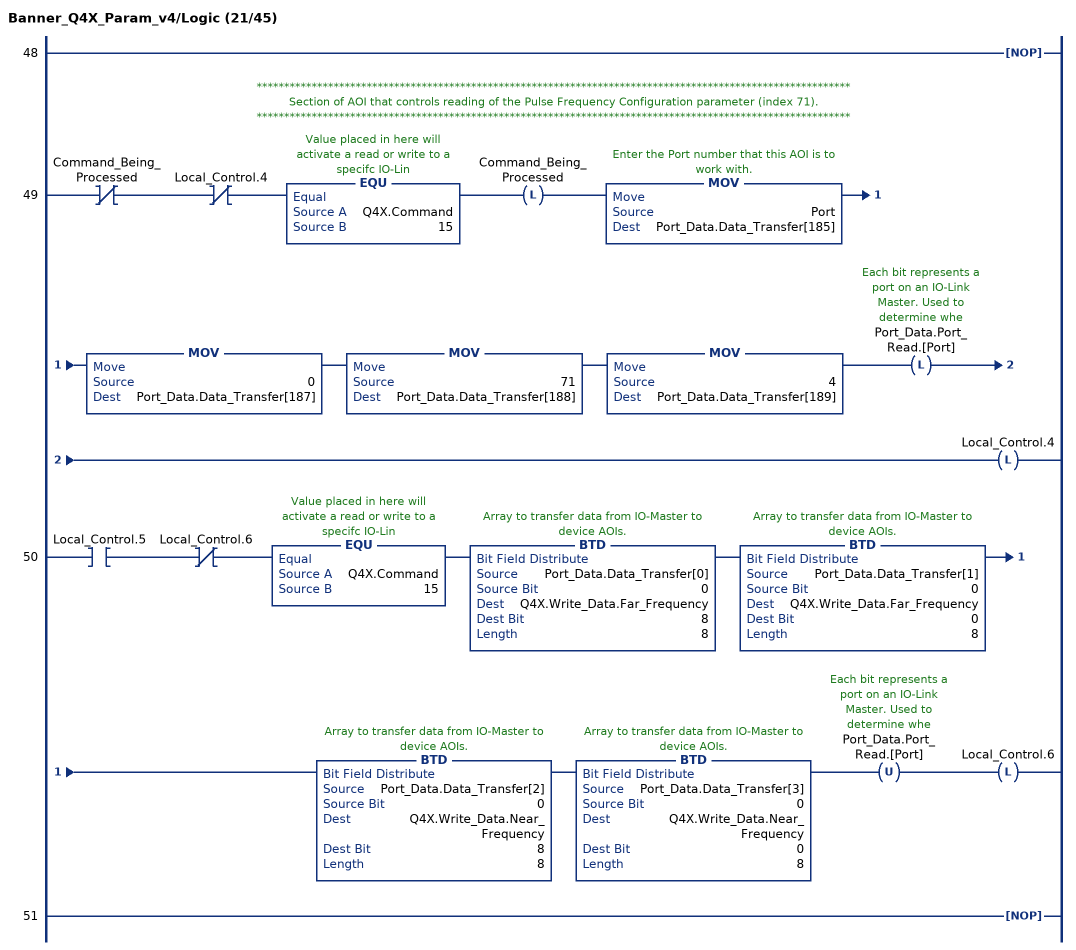
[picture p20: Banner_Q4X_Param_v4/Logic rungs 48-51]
   48: NOP();
   // ************************************************************************************************************
   // Section of AOI that controls reading of the Pulse Frequency Configuration parameter (index 71).
   // ************************************************************************************************************
   49: XIO(Command_Being_Processed)XIO(Local_Control.4)EQU(Q4X.Command,15)OTL(Command_Being_Processed)MOV(Port,Port_Data.Data_Transfer[185])MOV(0,Port_Data.Data_Transfer[187])MOV(71,Port_Data.Data_Transfer[188])MOV(4,Port_Data.Data_Transfer[189])OTL(Port_Data.Port_Read.[Port])OTL(Local_Control.4);
   50: XIC(Local_Control.5)XIO(Local_Control.6)EQU(Q4X.Command,15)BTD(Port_Data.Data_Transfer[0],0,Q4X.Write_Data.Far_Frequency,8,8)BTD(Port_Data.Data_Transfer[1],0,Q4X.Write_Data.Far_Frequency,0,8)BTD(Port_Data.Data_Transfer[2],0,Q4X.Write_Data.Near_Frequency,8,8)BTD(Port_Data.Data_Transfer[3],0,Q4X.Write_Data.Near_Frequency,0,8)OTU(Port_Data.Port_Read.[Port])OTL(Local_Control.6);
   51: NOP();
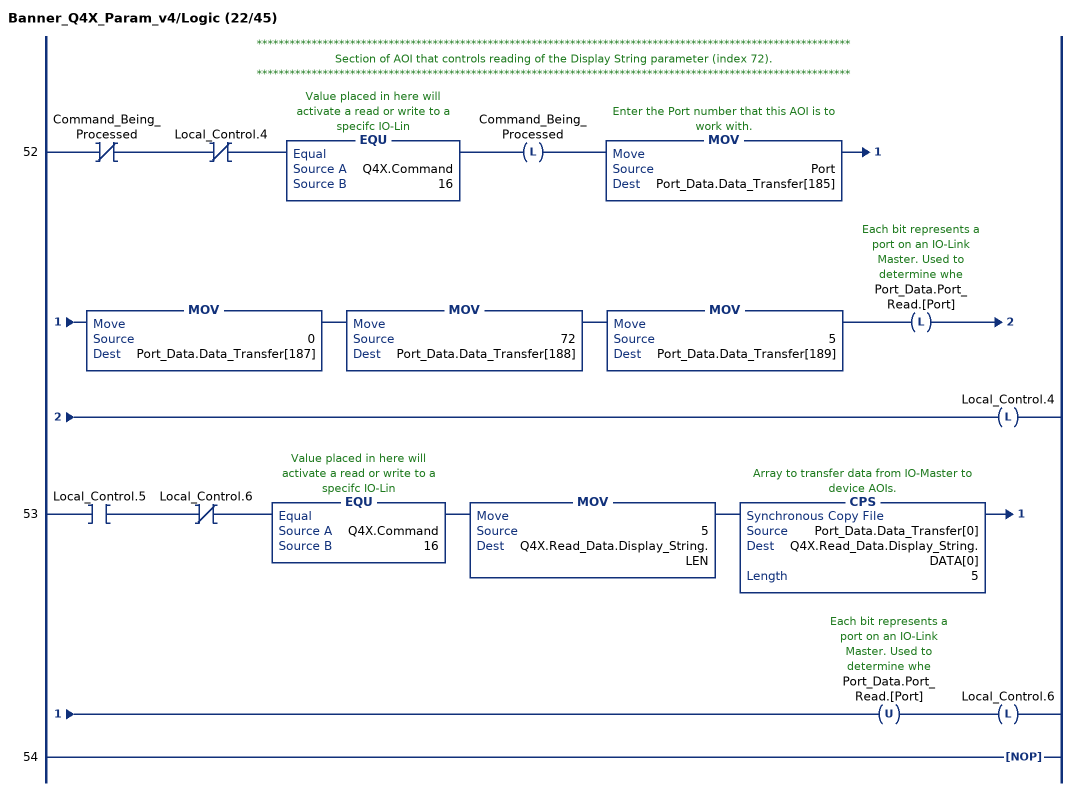
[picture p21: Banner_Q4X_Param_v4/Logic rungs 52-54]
   // ************************************************************************************************************
   // Section of AOI that controls reading of the Display String parameter (index 72).
   // ************************************************************************************************************
   52: XIO(Command_Being_Processed)XIO(Local_Control.4)EQU(Q4X.Command,16)OTL(Command_Being_Processed)MOV(Port,Port_Data.Data_Transfer[185])MOV(0,Port_Data.Data_Transfer[187])MOV(72,Port_Data.Data_Transfer[188])MOV(5,Port_Data.Data_Transfer[189])OTL(Port_Data.Port_Read.[Port])OTL(Local_Control.4);
   53: XIC(Local_Control.5)XIO(Local_Control.6)EQU(Q4X.Command,16)MOV(5,Q4X.Read_Data.Display_String.LEN)CPS(Port_Data.Data_Transfer[0],Q4X.Read_Data.Display_String.DATA[0],5)OTU(Port_Data.Port_Read.[Port])OTL(Local_Control.6);
   54: NOP();
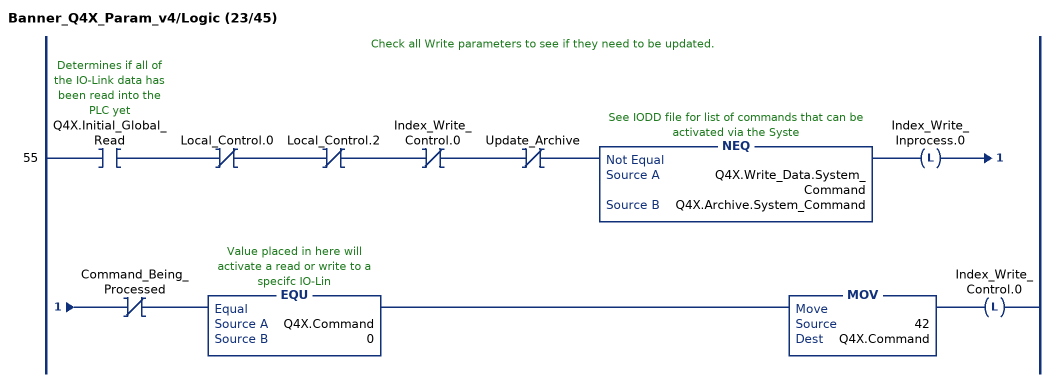
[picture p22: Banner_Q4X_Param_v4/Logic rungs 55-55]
   // Check all Write parameters to see if they need to be updated.
   55: XIC(Q4X.Initial_Global_Read)XIO(Local_Control.0)XIO(Local_Control.2)XIO(Index_Write_Control.0)XIO(Update_Archive)NEQ(Q4X.Write_Data.System_Command,Q4X.Archive.System_Command)OTL(Index_Write_Inprocess.0)XIO(Command_Being_Processed)EQU(Q4X.Command,0)MOV(42,Q4X.Command)OTL(Index_Write_Control.0);
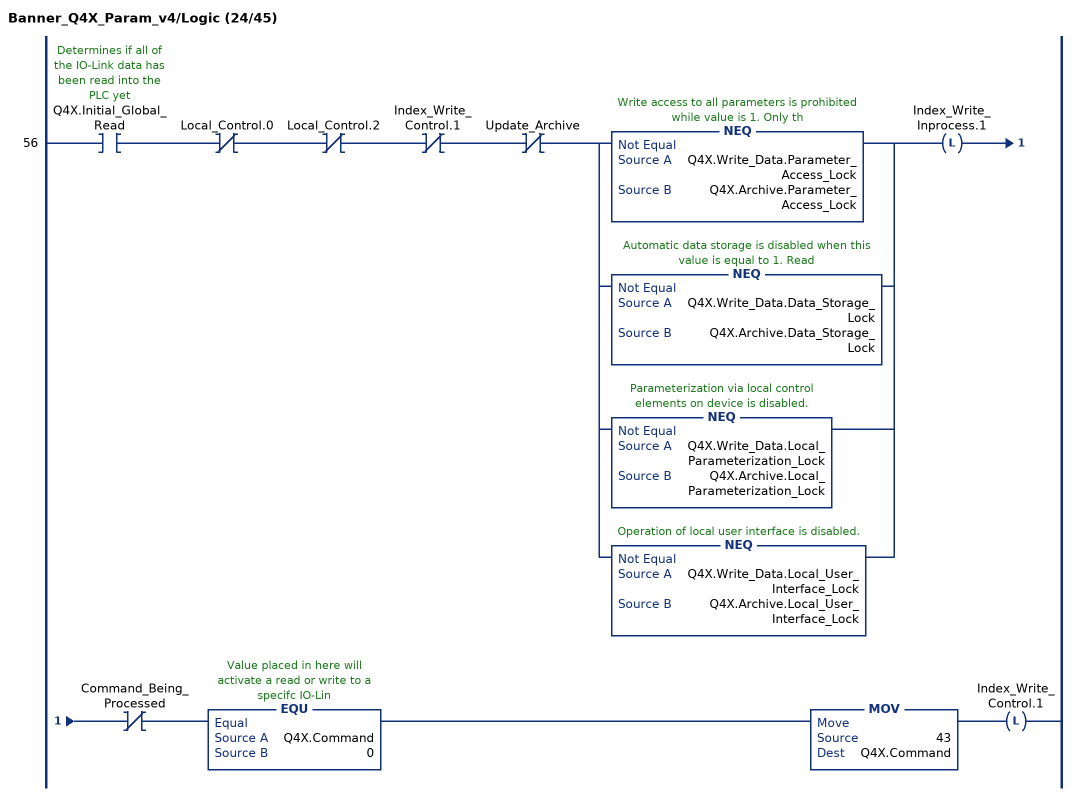
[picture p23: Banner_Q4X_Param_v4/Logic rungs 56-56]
   56: XIC(Q4X.Initial_Global_Read)XIO(Local_Control.0)XIO(Local_Control.2)XIO(Index_Write_Control.1)XIO(Update_Archive)[NEQ(Q4X.Write_Data.Parameter_Access_Lock,Q4X.Archive.Parameter_Access_Lock) ,NEQ(Q4X.Write_Data.Data_Storage_Lock,Q4X.Archive.Data_Storage_Lock) ,NEQ(Q4X.Write_Data.Local_Parameterization_Lock,Q4X.Archive.Local_Parameterization_Lock) ,NEQ(Q4X.Write_Data.Local_User_Interface_Lock,Q4X.Archive.Local_User_Interface_Lock) ]OTL(Index_Write_Inprocess.1)XIO(Command_Being_Processed)EQU(Q4X.Command,0)MOV(43,Q4X.Command)OTL(Index_Write_Control.1);
